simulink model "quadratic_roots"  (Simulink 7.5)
settings: Solver=VariableStepDiscrete  StartTime=0.0  StopTime=10.0  RelTol=1e-3

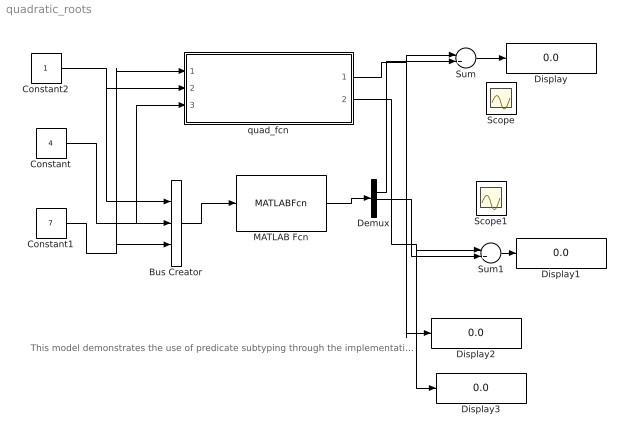
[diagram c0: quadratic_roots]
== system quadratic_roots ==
  note: This model demonstrates the use of predicate subtyping through the implementation of quad_fcn, which will give the real roots of a quadratic function. results are compared to the matlab function roots, results are generally the same, although sometimes there is a small error on the order of 1e-16. Currently does not activly check that inputs satisfy subtype constraints, in these cases proper output is not guaranteed. This example will not work under CVC3 as complex functions like sqrt are not supported.
  Bus Creator : BusCreator  Inputs=3
  Constant : Constant  Value=4  OutDataType=fixdt(1, 16)  OutScaling=2^0
  Constant1 : Constant  Value=7  OutDataType=fixdt(1, 16)  OutScaling=2^0
  Constant2 : Constant  OutDataType=fixdt(1, 16)  OutScaling=2^0
  Demux : Demux  Outputs=2
  Display{,1..3} (4 alike) : Display
  MATLAB Fcn : MATLABFcn  MATLABFcn=roots  OutputDimensions=2  Output1D=off
  Scope : Scope
  Scope1 : Scope
  Sum : Sum  Inputs=|+-  OutDataType=fixdt(1, 16)  OutScaling=2^0
  Sum1 : Sum  Inputs=|+-  OutDataType=fixdt(1, 16)  OutScaling=2^0
  quad_fcn : Subsystem
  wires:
  Constant2/1 -> Bus Creator/1, quad_fcn/2(a)
  Constant/1 -> Bus Creator/2, quad_fcn/3(b)
  Constant1/1 -> Bus Creator/3, quad_fcn/1(c)
  Bus Creator/1 -> MATLAB Fcn/1
  MATLAB Fcn/1 -> Demux/1
  quad_fcn/1(x1) -> Sum/1, Display2/1
  Demux/1 -> Sum/2
  Demux/2 -> Sum1/2
  quad_fcn/2(x2) -> Sum1/1, Display3/1
  Sum1/1 -> Display1/1
  Sum/1 -> Display/1

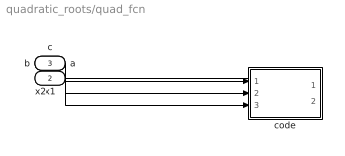
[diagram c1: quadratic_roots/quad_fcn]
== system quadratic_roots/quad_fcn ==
  c : Inport  OutDataType=fixdt(1, 16)  OutScaling=2^0
  a : Inport  Port=2  OutDataType=fixdt(1, 16)  OutScaling=2^0
  b : Inport  Port=3  OutDataType=fixdt(1, 16)  OutScaling=2^0
  code : Stateflow chart  TreatAsAtomicUnit=on
  x1 : Outport  OutDataType=fixdt(1, 16)  OutScaling=2^0
  x2 : Outport  Port=2  OutDataType=fixdt(1, 16)  OutScaling=2^0
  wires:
  c/1 -> code/1(c)
  a/1 -> code/2(a)
  b/1 -> code/3(b)
  code/1(x1) -> x1/1
  code/2(x2) -> x2/1

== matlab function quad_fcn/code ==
function [x1,x2] = quad_fcn(c,a,b)
%%#eml
x1=-c/b;
x2=-b/2*a;
if(a == 0)
  if(b ~= 0)
    x1 = -c/b;
    x2 = -c/b;
  end
elseif(a ~= 0)
  if((b^2) - 4*a*c == 0)
    x1 = -b/2*a;
    x2 = -b/2*a;
  elseif((b^2) - 4*a*c > 0)
    if(b>=0)
      x1 = (-b - sqrt(b^2 - 4*a*c)) / 2*a;
      x2 = c / (a* ((-b - sqrt(b^2 - 4*a*c)) / 2*a));
    elseif(b<0)
      x1 = (-b + sqrt(b^2 - 4*a*c)) / 2*a;
      x2 = c / (a* ((-b + sqrt(b^2 - 4*a*c)) / 2*a));
    end
  end
end
